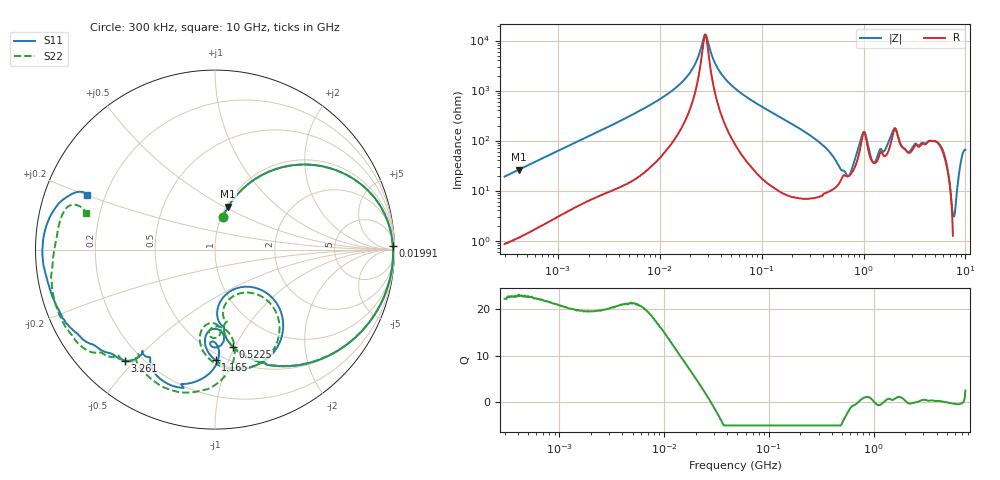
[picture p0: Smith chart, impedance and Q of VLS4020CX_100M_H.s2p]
! S-Parameter Data Generated by TDK Corporation
! Copyright(C) 2024 TDK Corporation.
! All Rights Reserved.
! TDK P/N: VLS4020CX-100M-H (SMD / SMT Inductor (Coil))
! Property: L=10uH at 1MHz
! Size(LxWxT): 4x4x2mm
! Model Type: s2p (Touchstone File Format Version 1.0)
! Frequency: DC=Yes Start=0.3MHz Stop=10000MHz 802points Log-sweep
! Model Generated on May 28, 2024
! Terms and conditions regarding TDK Simulation Models:
! 1)This simulation model is being provided solely for informational
!  purposes. Please refer to the specifications of the products in
!  terms of detailed characteristics of such products.
! 2)In no event shall TDK Corporation of any of its subsidiaries be
!  liable for any loss or damage arising, directly or indirectly,
!  from any information contained in this simulation model, including,
!  but not limited to loss or damages arising from any inaccuracies,
!  omissions or errors in connection with such information.
! 3)Any and all copyrights on this simulation model are owned by
!  TDK Corporation.  Duplication or redistribution of this simulation
!  model without prior written permission from TDK Corporation
!  is prohibited.
! 4)This simulation model is subject to any modification or change
!  without any prior notice.
! 5)Neither TDK Corporation nor any of its subsidiaries shall make any
!  warranty, express or implied, including but not limited to the
!  correctness, implied warranties of merchantability and fitness for
!  a particular purpose with respect to this simulation models.
! 6)The use of this simulation model shall be deemed to have consented
!  to the terms and conditions hereof.
! Port Assignments:
!  1 ---@@@--- 2
! Applicable Conditions:
!  Temperature = 25 degC
!  DC Bias Current = 0 A
!  Small Signal Operation
# Hz S MA R 50
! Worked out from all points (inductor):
!   801 points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, 300 kHz to 10 GHz, reference 50 ohm
!   read as one part in series: L = 10.1 uH near 318.3 kHz
!   highest Q = 22.8 at 415.4 kHz (marker M1), where L = 10.1 uH
!   self-resonance near 27.88 MHz
!   S11 on the Smith chart (normalised r, x): 300 kHz: 1.02, +0.38; 19.91 MHz: 38, +84; 522.5 MHz: 0.63, -0.99; 1.165 GHz: 0.45, -0.90; 3.261 GHz: 0.14, -0.47; 10 GHz: 0.13, +0.20
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300000  0.1848 76.6  0.9743 -10.8  0.9744 -10.7  0.1851 76.7
415395  0.2506 72.8  0.9571 -14.6  0.9571 -14.6  0.2508 72.9
1713600  0.7053 42.2  0.6735 -44.9  0.6737 -44.9  0.7053 42.2
9671944  0.9786 8.1  0.1519 -78.2  0.1519 -78.2  0.9787 8.1
1.990974e7  0.991 1.1  0.04278 -77.9  0.0428 -77.9  0.991 1.1
2.78833e7  0.9924 -1.8  0.007488 -4.4  0.007502 -4.4  0.9924 -1.7
3.729897e7  0.9922 -4.4  0.03645 74.5  0.03646 74.5  0.9923 -4.4
5.477226e7  0.9893 -8.6  0.08902 77.1  0.08904 77.1  0.9893 -8.5
1.540638e8  0.9394 -28.0  0.3139 60.2  0.3139 60.2  0.9393 -27.9
3.126428e8  0.7939 -54.3  0.5667 33.0  0.5668 33.0  0.7941 -54.0
5.225392e8  0.553 -79.5  0.7439 1.4  0.744 1.4  0.5506 -79.5
8.414386e8  0.2655 -51.1  0.7097 -48.3  0.7098 -48.3  0.3 -52.8
9.789263e8  0.6056 -51.8  0.3806 -60.5  0.3807 -60.5  0.6193 -55.9
1.165098e9  0.6168 -89.7  0.5158 -34.1  0.5161 -34.1  0.6069 -93.3
1.35547e9  0.4428 -91.7  0.6004 -60.7  0.6007 -60.8  0.4127 -94.6
1.767019e9  0.6052 -88.2  0.4199 -100.9  0.4198 -101.0  0.543 -78.6
2.08171e9  0.7957 -107.3  0.1883 -84.6  0.1883 -84.6  0.8104 -100.5
2.756092e9  0.6999 -125.4  0.2967 -95.5  0.2966 -95.6  0.7296 -126.5
3.261479e9  0.7961 -129.0  0.1857 -120.4  0.1855 -120.5  0.8015 -130.0
5.607117e9  0.9304 -155.7  0.06309 -119.5  0.06314 -119.6  0.9313 -150.0
7.222042e9  0.9596 -174.6  0.06195 -116.0  0.06174 -116.1  0.9258 -170.7
1e10  0.7738 156.9  0.05518 -124.1  0.05516 -124.0  0.745 164.0
